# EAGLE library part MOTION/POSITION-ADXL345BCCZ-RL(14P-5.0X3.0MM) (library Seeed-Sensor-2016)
314080008
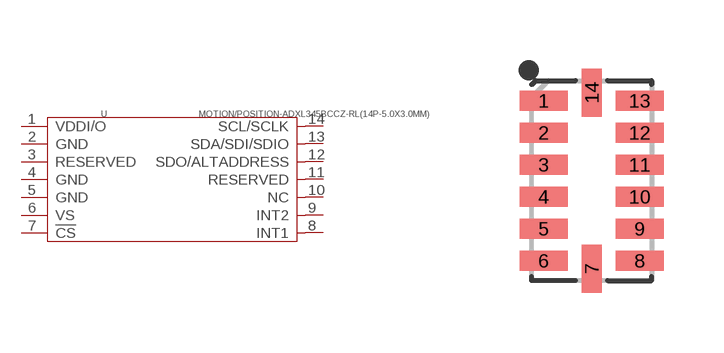
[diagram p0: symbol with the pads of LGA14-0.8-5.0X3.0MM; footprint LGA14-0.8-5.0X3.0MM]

Designator prefix U

## MOTION/POSITION-ADXL345BCCZ-RL(14P-5.0X3.0MM) (MPN: ADXL345BCCZ-RL; VALUE: ADXL345BCCZ-RL)  [LGA14-0.8-5.0X3.0MM]
1  VDDI/O  sup
2  GND  sup
3  RESERVED
4  GND  sup
5  GND  sup
6  VS
7  !CS
8  INT1
9  INT2
10  NC  nc
11  RESERVED
12  SDO/ALTADDRESS
13  SDA/SDI/SDIO
14  SCL/SCLK  in

## Footprint LGA14-0.8-5.0X3.0MM (pad centres in mm)
smd 1.2 x 0.5: 1 -1.2,2; 2 -1.2,1.2; 3 -1.2,0.4; 4 -1.2,-0.4; 5 -1.2,-1.2; 6 -1.2,-2; 8 1.2,-2; 9 1.2,-1.2; 10 1.2,-0.4; 11 1.2,0.4; 12 1.2,1.2; 13 1.2,2
smd 0.5 x 1.2: 7 0,-2.2; 14 0,2.2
